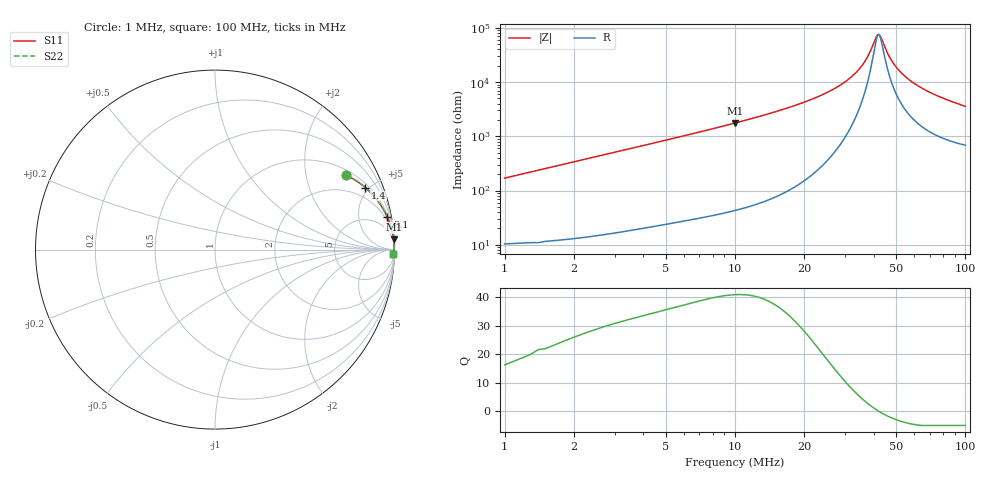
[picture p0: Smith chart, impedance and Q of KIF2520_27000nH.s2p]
!version-2
!date-12.2020
!Series
# MHz S RI R 50
!Freq ReS11 ImS11 ReS21 ImS21 ReS12 ImS12 ReS22 ImS22
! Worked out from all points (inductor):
!   991 points, 1 MHz to 100 MHz, reference 50 ohm
!   read as one part in series: L = 26.9 uH near 1.4 MHz
!   highest Q = 41 at 10 MHz (marker M1), where L = 28 uH
!   self-resonance near 42 MHz
!   S11 on the Smith chart (normalised r, x): 1 MHz: 1.21, +3.39; 1.4 MHz: 1.22, +4.75; 3.1 MHz: 1, +10; 100 MHz: 15, -70
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1  0.7301 0.4143  0.2699 -0.4143  0.2699 -0.4143  0.7301 0.4143
1.4  0.8383 0.3458  0.1617 -0.3458  0.1617 -0.3458  0.8383 0.3458
2.1  0.9186 0.2553  0.0814 -0.2553  0.0814 -0.2553  0.9186 0.2553
3.1  0.9595 0.1816  0.0405 -0.1816  0.0405 -0.1816  0.9595 0.1816
4.4  0.9787 0.1307  0.0213 -0.1307  0.0213 -0.1307  0.9787 0.1307
5.9  0.9876 0.098  0.0124 -0.098  0.0124 -0.098  0.9876 0.098
10  0.9954 0.0565  0.00459 -0.0565  0.00459 -0.0565  0.9954 0.0565
17.5  0.9983 0.0285  0.00167 -0.0285  0.00167 -0.0285  0.9983 0.0285
28  0.999 0.012  0.00104 -0.012  0.00104 -0.012  0.999 0.012
34  0.9989 0.00614  0.00108 -0.00614  0.00108 -0.00614  0.9989 0.00614
37.2  0.9988 0.00352  0.00116 -0.00352  0.00116 -0.00352  0.9988 0.00352
40.9  0.9987 0.000802  0.00128 -0.000802  0.00128 -0.000802  0.9987 0.000802
41.9  0.9987 0.000112  0.00132 -0.000112  0.00132 -0.000112  0.9987 0.000112
42.9  0.9986 -0.000562  0.00136 0.000562  0.00136 0.000562  0.9986 -0.000562
45.2  0.9985 -0.00205  0.00146 0.00205  0.00146 0.00205  0.9985 -0.00205
46.9  0.9985 -0.00311  0.00154 0.00311  0.00154 0.00311  0.9985 -0.00311
50.5  0.9983 -0.00524  0.00173 0.00524  0.00173 0.00524  0.9983 -0.00524
53.6  0.9981 -0.00696  0.00191 0.00696  0.00191 0.00696  0.9981 -0.00696
57.3  0.9979 -0.00892  0.00214 0.00892  0.00214 0.00892  0.9979 -0.00892
67  0.9972 -0.0136  0.00284 0.0136  0.00284 0.0136  0.9972 -0.0136
83.5  0.9957 -0.0208  0.0043 0.0208  0.0043 0.0208  0.9957 -0.0208
100  0.9939 -0.0271  0.00607 0.0271  0.00607 0.0271  0.9939 -0.0271
